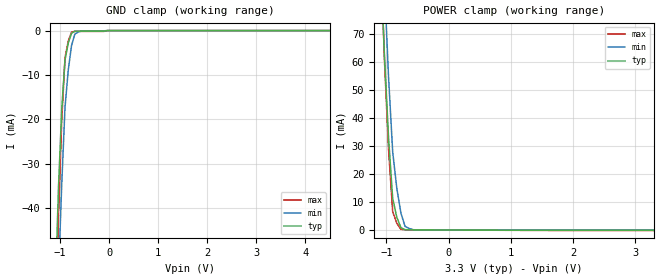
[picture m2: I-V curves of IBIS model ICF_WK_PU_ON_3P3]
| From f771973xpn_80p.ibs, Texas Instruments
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|   Model Cell ICF_WK_PU_ON_3P3
|ICF_WK_PU_ON_3P3
[Model]   ICF_WK_PU_ON_3P3
Model_type   Input
Polarity   Non-Inverting
Vinl =  0.8
Vinh =  2
C_comp   0.705929p   0.524756p   0.819798p
[Model Spec]
Vinl   0.8   0.8   0.8
Vinh   2   2   2
[Temperature Range]   25   155   -40
[Voltage Range]   3.3   2.97   3.63
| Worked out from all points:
|   GND clamp passes 1 mA (typ) near -0.78 V on its own axis
|   POWER clamp passes 1 mA (typ) near -0.77 V on its own axis
| Nom Voltages:
|   BIASFET=3.3, VDD=1.2, VDDS=3.3, VSS=0
| Min Voltages:
|   BIASFET=2.97, VDD=1.08, VDDS=2.97, VSS=0
| Max Voltages:
|   BIASFET=3.63, VDD=1.32, VDDS=3.63, VSS=0
[POWER_clamp]
|   voltage   I(typ)   I(min)   I(max)
-3.3V     1.823A     2.351A     1.96A
-1.1V     100.7mA    129.7mA    104mA
-1.033V   62.86mA    88.79mA    61.37mA
-966.7mV  33.07mA    54.88mA    28.9mA
-900mV    11.34mA    27.98mA    6.598mA
-833.3mV  4.564mA    14.87mA    2.388mA
-766.7mV  816.6uA    5.964mA    220.7uA
-700mV    102.1uA    1.265mA    96.3uA
-566.7mV  54.21uA    105.6uA    75.31uA
3.3V      -108.8uA   -51.5uA    -174uA
[GND_clamp]
|   voltage   I(typ)   I(min)   I(max)
-3.3V     -1.38A     -1.323A    -2.074A
-1.1V     -59.61mA   -79.12mA   -70.72mA
-1.033V   -35.5mA    -55.25mA   -41.84mA
-966.7mV  -17.84mA   -34.66mA   -20.33mA
-900mV    -6.616mA   -17.33mA   -6.173mA
-833.3mV  -2.77mA    -8.87mA    -2.348mA
-766.7mV  -612.2uA   -3.359mA   -349.7uA
-700mV    -142uA     -800.2uA   -179.5uA
-566.7mV  -110.1uA   -110.9uA   -175.3uA
-500mV    -109.3uA   -59.84uA   -175.2uA
-33.33mV  0A         0A         0A
6.6V      0A         0A         0A
